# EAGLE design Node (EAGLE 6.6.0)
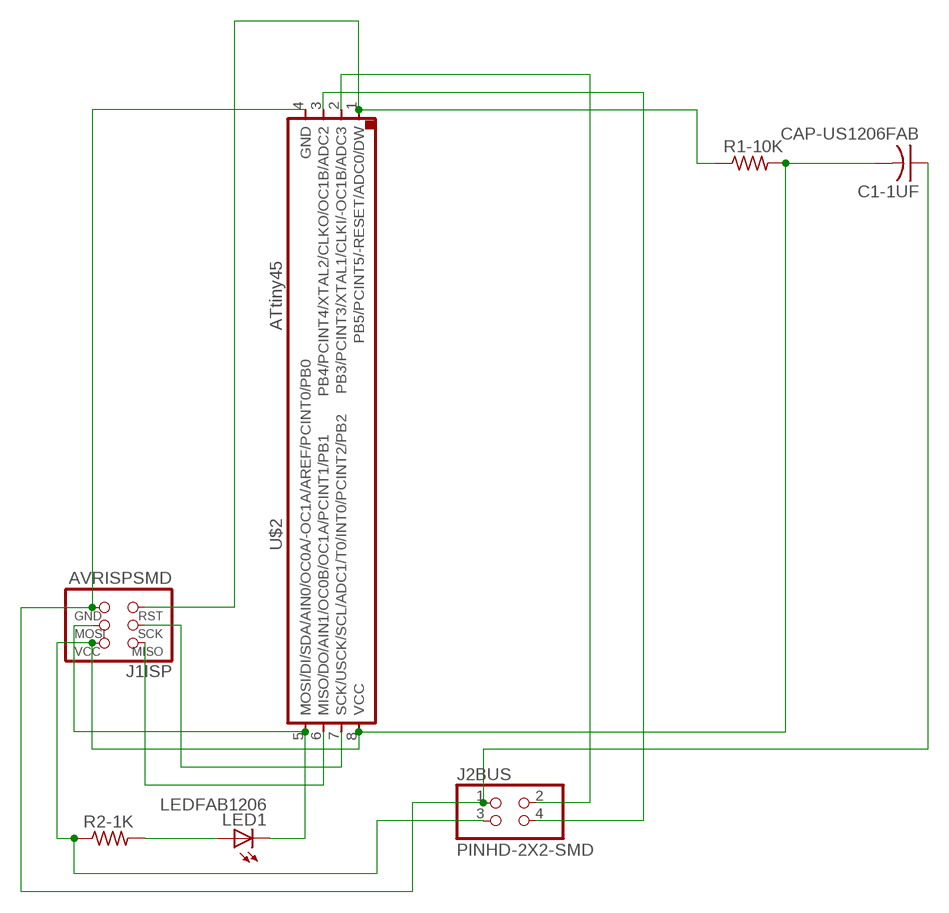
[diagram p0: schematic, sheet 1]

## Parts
C1-1UF  CAP-US1206FAB  [C1206FAB]
J1ISP  AVRISPSMD  [2X03SMD]
J2BUS  PINHD-2X2-SMD  [2X02SMD]
LED1  LEDFAB1206  [LED1206FAB]
R1-10K  RES-US1206FAB  [R1206FAB]
R2-1K  RES-US1206FAB  [R1206FAB]
U$2  ATTINY45SI  [SOIC8]

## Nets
N$1: C1-1UF.2 J1ISP.2(VCC) J2BUS.3 R1-10K.2 R2-1K.1 U$2.8(VCC)
N$3: J1ISP.3(SCK) U$2.7(SCK/USCK/SCL/ADC1/T0/INT0/PCINT2/PB2)
N$4: J1ISP.1(MISO) U$2.6(MISO/DO/AIN1/OC0B/OC1A/PCINT1/PB1)
N$5: J1ISP.4(MOSI) LED1.2(C) U$2.5(MOSI/DI/SDA/AIN0/OC0A/-OC1A/AREF/PCINT0/PB0)
N$6: C1-1UF.1 J1ISP.6(GND) J2BUS.1 U$2.4(GND)
N$7: J2BUS.4 U$2.3(PB4/PCINT4/XTAL2/CLKO/OC1B/ADC2)
N$8: J2BUS.2 U$2.2(PB3/PCINT3/XTAL1/CLKI/-OC1B/ADC3)
N$9: J1ISP.5(RST) R1-10K.1 U$2.1(PB5/PCINT5/-RESET/ADC0/DW)
N$10: LED1.1(A) R2-1K.2

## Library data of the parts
C1-1UF = fab:CAP-US
J1ISP = fab:AVRISP
J2BUS = fab:PINHD-2X2-SMD
LED1 = fab:LED: LED
R1-10K R2-1K = fab:RES-US: Resistor (US Symbol)
U$2 = fab:ATTINY45

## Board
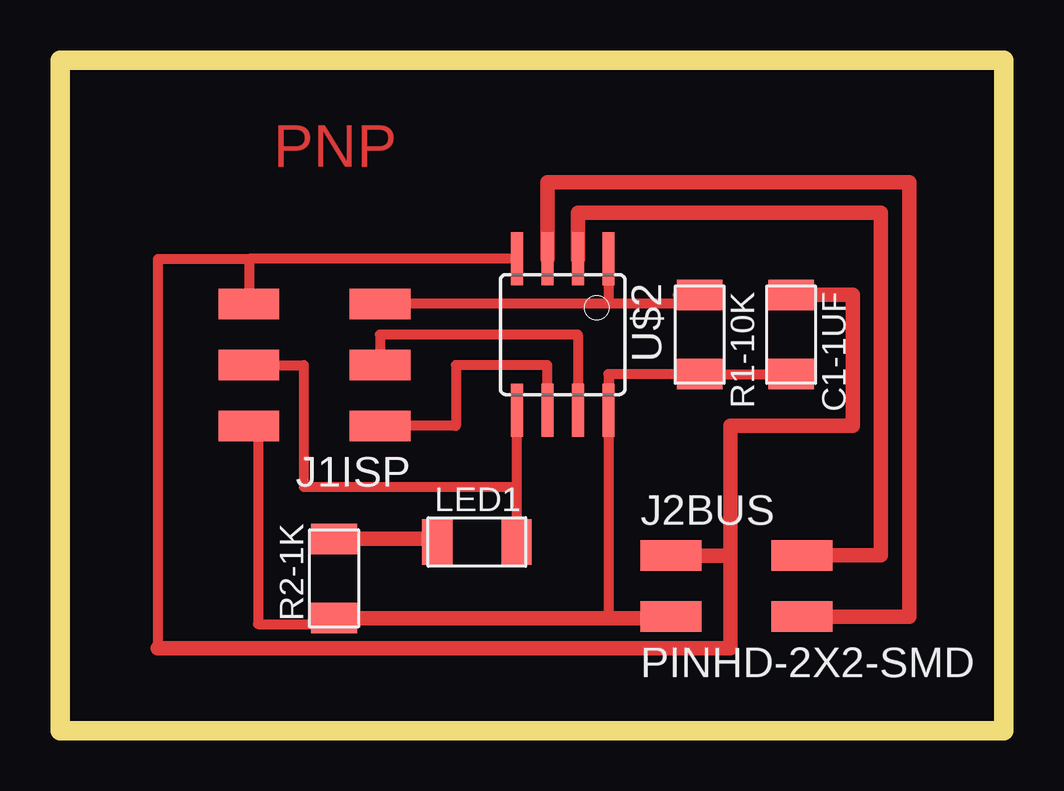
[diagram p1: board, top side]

Size 39.35 x 27.95 mm. Coordinates in mm from the lower left corner, seen from the top.
Outline: 0,0 39.35,0 39.35,27.95 0,27.95 0,0
Copper layers (1*16): Top 0.035mm / dielectric 1.5mm / Bottom 0.035mm
Design rules "default": minimum track width 10mil, minimum drill 24mil, track to track 8mil, track to pad 8mil, pad to pad 8mil, via to via 8mil, smd to smd 8mil, copper to edge 40mil, drill to drill 8mil, minimum pad ring 10mil, minimum via ring 8mil, stop-mask expansion 4mil, vias tented up to drill 0mil, thermal gap 10mil

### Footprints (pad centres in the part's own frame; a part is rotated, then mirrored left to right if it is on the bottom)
C1206FAB = smd 1.27 x 1.905: 1 -1.651,0; 2 1.651,0
2X03SMD = smd 2.54 x 1.27: 1 -2.54,2.54; 2 2.92,2.54; 3 -2.54,0; 4 2.92,0; 5 -2.54,-2.54; 6 2.92,-2.54
2X02SMD = smd 2.54 x 1.27: 1 -2.54,1.27; 2 2.92,1.27; 3 -2.54,-1.27; 4 2.92,-1.27
LED1206FAB = smd 1.27 x 1.905: 1 -1.651,0; 2 1.651,0
R1206FAB = smd 1.27 x 1.905: 1 -1.651,0; 2 1.651,0
SOIC8 = smd 0.5 x 2.2: 1 -1.905,-3.154; 2 -0.645,-3.154; 3 0.625,-3.154; 4 1.895,-3.154; 5 1.905,3.154; 6 0.635,3.154; 7 -0.635,3.154; 8 -1.905,3.154

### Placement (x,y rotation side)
C1-1UF  30.48,16.51 270 top
J1ISP  10.79,15.24 180 top
J2BUS  28,6.03 0 top
LED1  17.38,7.87 0 top
R1-10K  26.67,16.51 270 top
R2-1K  11.43,6.35 90 top
U$2  20.95,16.51 180 top

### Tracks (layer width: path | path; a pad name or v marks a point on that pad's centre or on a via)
N$1
  Top 0.406: U$2.8 22.91,13.36 22.91,14.86 | 22.91,14.86 R1-10K.2 C1-1UF.2 | 22.91,14.86 22.86,14.86 22.86,4.7 | J1ISP.2 8.26,12.7 8.26,4.45 11.43,4.45 R2-1K.1
  Top 0.61: R2-1K.1 22.86,4.7 25.4,4.7 J2BUS.3
N$3
  Top 0.406: U$2.7 21.59,16.51 13.34,16.51 J1ISP.3
N$4
  Top 0.406: U$2.6 20.32,15.24 16.51,15.24 16.51,12.7 J1ISP.1
N$5
  Top 0.406: 19.03,10.16 10.16,10.16 10.16,15.24 J1ISP.4 | U$2.5 19.05,10.16 19.03,10.16 | 19.03,10.16 LED1.2
N$6
  Top 0.406: U$2.4 7.88,19.66 | 4.07,3.43 4.07,19.66 7.88,19.66 | 7.88,19.66 J1ISP.6
  Top 0.61: J2BUS.1 27.94,7.3 | 27.94,7.3 27.94,12.7 33.04,12.7 33.04,18.18 30.48,18.18 C1-1UF.1 | 4.07,3.43 27.94,3.43 27.94,7.3
N$7
  Top 0.61: U$2.3 20.32,22.86 35.41,22.86 35.41,4.76 J2BUS.4
N$8
  Top 0.61: U$2.2 21.59,21.59 34.23,21.59 34.23,7.32 30.92,7.32 J2BUS.2
N$9
  Top 0.406: R1-10K.1 25.75,18.16 25.75,17.8 22.86,17.8 | 22.86,17.8 13.34,17.8 J1ISP.5 | U$2.1 22.86,17.8
N$10
  Top 0.61: R2-1K.2 15.73,8 LED1.1

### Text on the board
Top: PNP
